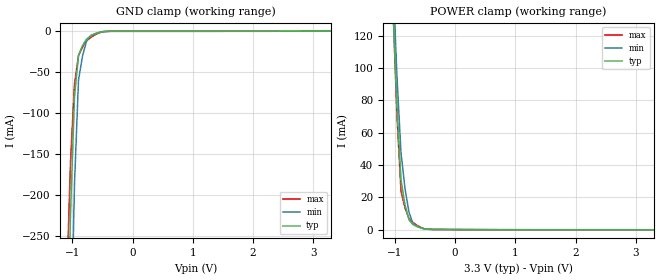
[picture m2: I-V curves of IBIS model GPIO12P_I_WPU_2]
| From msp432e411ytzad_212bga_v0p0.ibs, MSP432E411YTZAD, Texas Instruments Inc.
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|   Model Cell GPIO12P_I_WPU_2
[Model]   GPIO12P_I_WPU_2
Model_type   Input
Polarity   Non-Inverting
Vinl =  0.8
Vinh =  2
C_comp   6.029616p   5.226915p   6.778838p
[Model Spec]
Vinl   0.8   0.8   0.8
Vinh   2   2   2
[Temperature Range]   25   125   -40
[Voltage Range]   3.3   2.97   3.63
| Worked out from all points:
|   GND clamp passes 1 mA (typ) near -0.52 V on its own axis
|   POWER clamp passes 1 mA (typ) near -0.57 V on its own axis
| Nom Voltages:
|   IBIASFET=3.3, VDDC=1.2, VDD=3.3, GND=0
| Min Voltages:
|   IBIASFET=2.97, VDDC=1.08, VDD=2.97, GND=0
| Max Voltages:
|   IBIASFET=3.63, VDDC=1.32, VDD=3.63, GND=0
[POWER_clamp]
|   voltage   I(typ)   I(min)   I(max)
-3.3V     3.668A     4.187A     4.057A
-1.033V   137.2mA    154.8mA    137.3mA
-966.7mV  76.02mA    94.43mA    70.06mA
-900mV    30.7mA     47.61mA    23.73mA
-833.3mV  15.22mA    25.33mA    13.29mA
-766.7mV  6.012mA    10.62mA    6.847mA
-700mV    3.066mA    3.493mA    4.387mA
-566.7mV  916.3uA    905.1uA    1.247mA
-500mV    288.8uA    338.8uA    340.1uA
-366.7mV  64.4uA     61.42uA    82.87uA
3.3V      -165.6uA   -105.9uA   -263uA
[GND_clamp]
|   voltage   I(typ)   I(min)   I(max)
-3.3V     -18.01A    -17.27A    -18.6A
-1.1V     -459.9mA   -734.3mA   -318.7mA
-1.033V   -223.6mA   -411.6mA   -160.4mA
-966.7mV  -80.12mA   -186.8mA   -64.22mA
-900mV    -29.52mA   -59.81mA   -30.12mA
-833.3mV  -17.68mA   -30.41mA   -19.46mA
-766.7mV  -9.826mA   -12.3mA    -12.05mA
-700mV    -5.959mA   -5.476mA   -7.887mA
-500mV    -638.9uA   -656.2uA   -802.2uA
-366.7mV  -189uA     -142.2uA   -285.7uA
3.3V      65.25pA    38.54uA    -61.41uA
